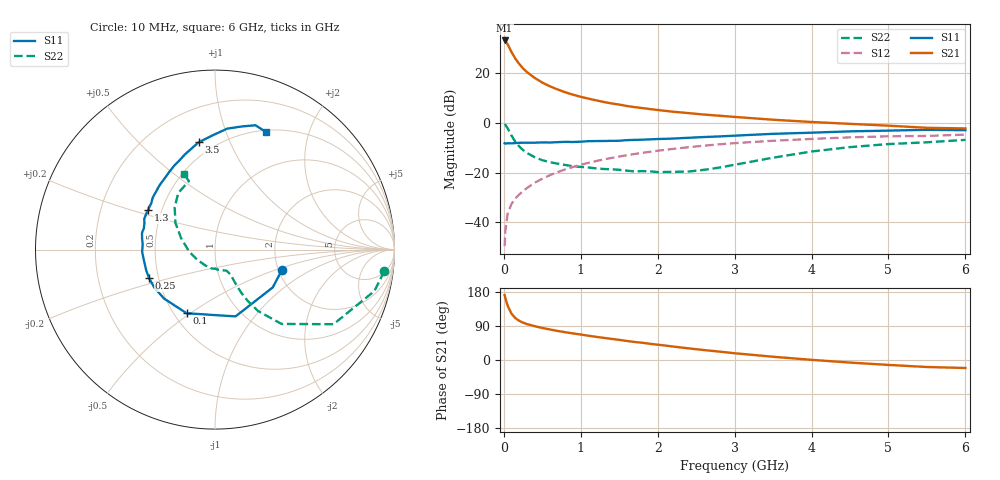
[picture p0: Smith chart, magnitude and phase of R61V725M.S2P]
! SIEMENS Small Signal Semiconductors
! BFR193
! Si NPN RF Bipolar Junction Transistor in SOT23
! VCE = 1.75 V  IC = 25 mA
! Common Emitter S-Parameters:  May  1996
# GHz  S  MA  R  50
!  f  S11  S21  S12  S22
! GHz  MAG  ANG  MAG  ANG  MAG  ANG  MAG  ANG
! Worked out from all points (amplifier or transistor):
!   36 points, 10 MHz to 6 GHz, reference 50 ohm
!   highest |S21| = 33.2 dB at 10 MHz (marker M1)
!   |S21| within 3 dB of that: start of sweep to 72.45 MHz
!   unconditionally stable (mu >= 1): 472.8 MHz to 1.945 GHz
!   at 250 MHz: K = 0.89, MSG = 24.7 dB, |S12| = -27.5 dB
!   at 1.4 GHz: K = 1.03, MAG = 10.0 dB, |S12| = -14.1 dB
!   at 6 GHz: K = 0.96, MSG = 1.2 dB, |S12| = -4.7 dB
!   S11 on the Smith chart (normalised r, x): 10 MHz: 2.09, -0.56; 100 MHz: 0.58, -0.48; 250 MHz: 0.44, -0.17; 1.3 GHz: 0.42, +0.23; 3.5 GHz: 0.41, +0.77; 6 GHz: 0.52, +1.39
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0.01  0.3897 -17.0  45.95 171.5  0.0033 84.4  0.951 -7.3
0.02  0.3846 -33.2  44.8 163.1  0.0067 80.8  0.9173 -14.6
0.05  0.3894 -72.9  38.11 142.8  0.0151 69.5  0.7801 -32.2
0.1  0.3883 -114.0  26.78 122.2  0.0235 63.8  0.5556 -48.2
0.15  0.3936 -136.0  19.73 110.4  0.0303 63.8  0.4173 -55.0
0.2  0.3989 -147.8  15.46 103.5  0.0364 65.3  0.3376 -57.5
0.25  0.4003 -156.4  12.56 98.5  0.0423 66.6  0.2843 -58.6
0.3  0.4003 -163.2  10.61 94.8  0.0489 68.3  0.2491 -58.8
0.4  0.4011 -172.3  8.101 89.3  0.0625 69.8  0.205 -58.7
0.5  0.406 -178.2  6.514 84.6  0.0752 70.2  0.1778 -58.2
0.6  0.4039 175.9  5.468 80.5  0.089 70.0  0.1623 -58.3
0.7  0.4109 171.3  4.726 76.6  0.1025 69.8  0.1515 -59.2
0.8  0.4172 167.1  4.153 73.3  0.1166 69.1  0.1422 -60.3
0.9  0.414 163.3  3.706 70.1  0.1304 68.3  0.1345 -61.5
1.1  0.43 156.5  3.093 64.1  0.1573 66.1  0.127 -66.6
1.3  0.4333 149.4  2.646 58.4  0.1845 63.8  0.1182 -72.6
1.7  0.4565 137.7  2.085 47.5  0.2372 58.4  0.1057 -89.8
2.2  0.485 125.6  1.686 35.5  0.3008 51.1  0.1036 -120.3
3.5  0.6047 98.7  1.163 8.6  0.438 30.7  0.2001 161.1
4.5  0.6777 84.2  0.96 -6.8  0.5131 16.4  0.3263 133.5
5.5  0.7284 72.0  0.799 -18.5  0.5486 2.4  0.4082 110.9
6  0.7147 66.7  0.777 -21.1  0.5835 -1.7  0.4564 112.3
